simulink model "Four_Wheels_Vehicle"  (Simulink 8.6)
settings: Solver=ode45  StartTime=0.0  StopTime=20  RelTol=1e-3
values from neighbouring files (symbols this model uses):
  beta = 1    [Vehicle_Parameters.m]
  g = 9.81    [Vehicle_Parameters.m]
  H_CoG = 0.700    (= 0.7)    [Vehicle_Parameters.m]
  Hearo = 0.750    (= 0.75)    [Vehicle_Parameters.m]
  Iz = 2480    [Vehicle_Parameters.m]
  Jw = 2.166    [Vehicle_Parameters.m]
  L = 10    [Vehicle_Parameters.m]
  Lf = 1.180    (= 1.18)    [Vehicle_Parameters.m]
  Lr = 1.770    (= 1.77)    [Vehicle_Parameters.m]
  Lw = 1.880    (= 1.88)    [Vehicle_Parameters.m]
  m = 1500    [Vehicle_Parameters.m]
  miu = 0.85    [Vehicle_Parameters.m]
  reff = 0.380    (= 0.38)    [Vehicle_Parameters.m]
undefined symbols (not defined in the file or in its folder): DiscIntNeverNeededParam, Init, Ki, Kp, LowerLimit, sigbuilder_block, Ts, UpperLimit
libraries: simulink x15, powerlib_extras x3
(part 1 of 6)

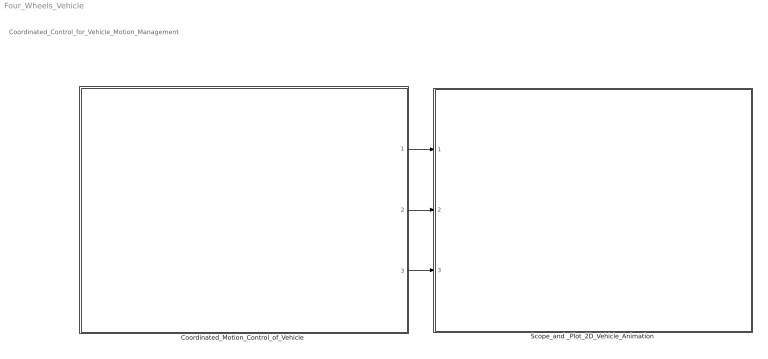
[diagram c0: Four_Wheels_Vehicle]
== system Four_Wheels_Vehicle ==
  note: Coordinated_Control_for_Vehicle_Motion_Management
  "Coordinated_Motion_Control_of_Vehicle " : Subsystem
  Scope_and _Plot_2D_Vehicle_Animation : Subsystem
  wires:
  "Coordinated_Motion_Control_of_Vehicle "/2(Control_of_braking_without_steering_control) -> Scope_and _Plot_2D_Vehicle_Animation/2(Control_of_braking_without_steering_control)
  "Coordinated_Motion_Control_of_Vehicle "/1(Coordinated_motion_control_Steering+Braking) -> Scope_and _Plot_2D_Vehicle_Animation/1(Coordinated_motion_control_Steering+Braking)
  "Coordinated_Motion_Control_of_Vehicle "/3(Control_of_steering_without_braking_control) -> Scope_and _Plot_2D_Vehicle_Animation/3(Control_of_steering_without_braking_control)

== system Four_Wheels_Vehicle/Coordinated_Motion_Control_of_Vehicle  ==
  Control_of_braking_without_steering_control. : Subsystem
  Control_of_steering_without_braking_control. : Subsystem
  Coordinated_motion_control_Steering+Braking. : Subsystem
  Mux : Mux  Inputs=8
  Mux1 : Mux  Inputs=8
  Mux2 : Mux  Inputs=8
  Coordinated_motion_control_Steering+Braking : Outport
  Control_of_braking_without_steering_control : Outport  Port=2
  Control_of_steering_without_braking_control : Outport  Port=3
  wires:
  Mux/1 -> Coordinated_motion_control_Steering+Braking/1
  Coordinated_motion_control_Steering+Braking./8(Ideal) -> Mux/8
  Coordinated_motion_control_Steering+Braking./6(yaw_pos.) -> Mux/6
  Coordinated_motion_control_Steering+Braking./7(SteeringAng) -> Mux/7
  Coordinated_motion_control_Steering+Braking./5(y_Vel) -> Mux/5
  Coordinated_motion_control_Steering+Braking./4(x_Vel) -> Mux/4
  Coordinated_motion_control_Steering+Braking./3(Tyre_speed) -> Mux/3
  Coordinated_motion_control_Steering+Braking./2(Estimated_trajectory) -> Mux/2
  Coordinated_motion_control_Steering+Braking./1(Ideal_trajectory) -> Mux/1
  Control_of_braking_without_steering_control./1(Ideal_trajectory_1) -> Mux1/1
  Control_of_braking_without_steering_control./2(Estimated_trajectory_1) -> Mux1/2
  Control_of_braking_without_steering_control./4(x_Vel_1) -> Mux1/4
  Control_of_braking_without_steering_control./5(y_Vel_1) -> Mux1/5
  Control_of_braking_without_steering_control./6(yaw_pos_1) -> Mux1/6
  Control_of_braking_without_steering_control./7(SteeringAng_1) -> Mux1/7
  Control_of_braking_without_steering_control./8(Ideal_1) -> Mux1/8
  Mux1/1 -> Control_of_braking_without_steering_control/1
  Control_of_steering_without_braking_control./1(Ideal_trajectory) -> Mux2/1
  Control_of_steering_without_braking_control./2(Estimated_trajectory) -> Mux2/2
  Control_of_steering_without_braking_control./3(Tyre_speed) -> Mux2/3
  Control_of_steering_without_braking_control./4(x_Vel) -> Mux2/4
  Control_of_steering_without_braking_control./5(y_Vel) -> Mux2/5
  Control_of_steering_without_braking_control./6(yaw_pos_2) -> Mux2/6
  Control_of_steering_without_braking_control./7(SteeringAng) -> Mux2/7
  Control_of_steering_without_braking_control./8(Ideal) -> Mux2/8
  Mux2/1 -> Control_of_steering_without_braking_control/1
  Control_of_braking_without_steering_control./3(Tyre_speed_1) -> Mux1/3

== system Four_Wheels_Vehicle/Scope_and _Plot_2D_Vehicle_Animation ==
  Coordinated_motion_control_Steering+Braking : Inport
  Control_of_braking_without_steering_control : Inport  Port=2
  Control_of_steering_without_braking_control : Inport  Port=3
  Scope_and _Plot_2D_Vehicle_Animation : Subsystem
  Signal_arrangement : Subsystem
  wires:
  Coordinated_motion_control_Steering+Braking/1 -> Signal_arrangement/1(Coordinated_motion_control_Steering+Braking)
  Control_of_braking_without_steering_control/1 -> Signal_arrangement/2(Control_of_braking_without_steering_control)
  Control_of_steering_without_braking_control/1 -> Signal_arrangement/3(Control_of_steering_without_braking_control)
  Signal_arrangement/1(Ideal_trajectory) -> Scope_and _Plot_2D_Vehicle_Animation/1(Ideal_trajectory)
  Signal_arrangement/2(Estimated_trajectory) -> Scope_and _Plot_2D_Vehicle_Animation/2(Estimated_trajectory)
  Signal_arrangement/3(Speed) -> Scope_and _Plot_2D_Vehicle_Animation/3(Speed)
  Signal_arrangement/4(Ideal_trajectory_1) -> Scope_and _Plot_2D_Vehicle_Animation/4(Ideal_trajectory_1)
  Signal_arrangement/5(Estimated_trajectory_1) -> Scope_and _Plot_2D_Vehicle_Animation/5(Estimated_trajectory_1)
  Signal_arrangement/6(Speed_1) -> Scope_and _Plot_2D_Vehicle_Animation/6(Speed_1)
  Signal_arrangement/7(Ideal_trajectory_2) -> Scope_and _Plot_2D_Vehicle_Animation/7(Ideal_trajectory_2)
  Signal_arrangement/8(Estimated_trajectory_2) -> Scope_and _Plot_2D_Vehicle_Animation/8(Estimated_trajectory_2)
  Signal_arrangement/9(Speed_2) -> Scope_and _Plot_2D_Vehicle_Animation/9(Speed_2)

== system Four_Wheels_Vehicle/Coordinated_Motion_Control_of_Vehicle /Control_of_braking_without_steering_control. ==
  note: Control_of_braking_without_steering_control
  Driver_command_1 : Subsystem
  Full_Vehicle_and_Tyre_Models_1 : Subsystem
  Motion_Coordinator_1 : Subsystem
  Scopes_and_2Dvehicle_1 : Subsystem
  Ideal_trajectory_1 : Outport
  Estimated_trajectory_1 : Outport  Port=2
  Tyre_speed_1 : Outport  Port=3
  x_Vel_1 : Outport  Port=4
  y_Vel_1 : Outport  Port=5
  yaw_pos_1 : Outport  Port=6
  SteeringAng_1 : Outport  Port=7
  Ideal_1 : Outport  Port=8
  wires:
  Motion_Coordinator_1/1(Ideal_traj._1) -> Scopes_and_2Dvehicle_1/2(Ideal._1)
  Scopes_and_2Dvehicle_1/8(Ideal_1) -> Ideal_1/1
  Scopes_and_2Dvehicle_1/7(SteeringAng_1) -> SteeringAng_1/1
  Scopes_and_2Dvehicle_1/5(y_Vel_1) -> y_Vel_1/1
  Scopes_and_2Dvehicle_1/4(x_Vel_1) -> x_Vel_1/1
  Scopes_and_2Dvehicle_1/2(Estimated_trajectory_1) -> Estimated_trajectory_1/1
  Scopes_and_2Dvehicle_1/1(Ideal_trajectory_1) -> Ideal_trajectory_1/1
  Driver_command_1/1(Steering_Ang._1) -> Motion_Coordinator_1/1(Steering_Ang_1), Scopes_and_2Dvehicle_1/1(SteeringAng._1)
  Full_Vehicle_and_Tyre_Models_1/2(x_Vel_1) -> Scopes_and_2Dvehicle_1/4(x_Vel._1), Motion_Coordinator_1/2(x_Vel)
  Full_Vehicle_and_Tyre_Models_1/5(yaw_rate_1) -> Motion_Coordinator_1/4(yaw_feedback_1), Scopes_and_2Dvehicle_1/7(yaw_rate._1)
  Full_Vehicle_and_Tyre_Models_1/4(sideslip_angle_1) -> Motion_Coordinator_1/3(Sideslip_feedback_1), Scopes_and_2Dvehicle_1/6(sideslipAng_1)
  Motion_Coordinator_1/2(f_1) -> Full_Vehicle_and_Tyre_Models_1/1(SteeringAng_1)
  Motion_Coordinator_1/3(Mzc_all_1) -> Full_Vehicle_and_Tyre_Models_1/2(Mzc_all_1)
  Full_Vehicle_and_Tyre_Models_1/3(y_Vel_1) -> Scopes_and_2Dvehicle_1/5(y_Vel._1)
  Motion_Coordinator_1/4(yaw_pos._1) -> yaw_pos_1/1
  Full_Vehicle_and_Tyre_Models_1/1(Tyre_speed_1) -> Scopes_and_2Dvehicle_1/3(Tyre_speed_1)
  Scopes_and_2Dvehicle_1/3(Tyre_speed_1.) -> Tyre_speed_1/1

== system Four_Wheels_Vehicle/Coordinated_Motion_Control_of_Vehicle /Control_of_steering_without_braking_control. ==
  note: Control_of_steering_without_braking_control
  Driver_command_2 : Subsystem
  Full_Vehicle_and_Tyre_Models_2 : Subsystem
  Motion_Coordinator_2 : Subsystem
  Scopes_and_2Dvehicle_2 : Subsystem
  Ideal_trajectory : Outport
  Estimated_trajectory : Outport  Port=2
  Tyre_speed : Outport  Port=3
  x_Vel : Outport  Port=4
  y_Vel : Outport  Port=5
  yaw_pos_2 : Outport  Port=6
  SteeringAng : Outport  Port=7
  Ideal : Outport  Port=8
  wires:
  Driver_command_2/1(Steering_Ang._2) -> Scopes_and_2Dvehicle_2/1(SteeringAng._2), Motion_Coordinator_2/1(Steering_Ang_2)
  Scopes_and_2Dvehicle_2/1(Ideal_trajectory_2) -> Ideal_trajectory/1
  Scopes_and_2Dvehicle_2/2(Estimated_trajectory_2) -> Estimated_trajectory/1
  Scopes_and_2Dvehicle_2/4(x_Vel_2) -> x_Vel/1
  Scopes_and_2Dvehicle_2/5(y_Vel_2) -> y_Vel/1
  Scopes_and_2Dvehicle_2/7(SteeringAng_2) -> SteeringAng/1
  Scopes_and_2Dvehicle_2/8(Ideal_2) -> Ideal/1
  Motion_Coordinator_2/1(Ideal_traj._2) -> Scopes_and_2Dvehicle_2/2(Ideal._2)
  Full_Vehicle_and_Tyre_Models_2/5(sideslip_angle) -> Motion_Coordinator_2/4(Sideslip_feedback_2), Scopes_and_2Dvehicle_2/7(sideslipAng_2)
  Full_Vehicle_and_Tyre_Models_2/4(yaw_rate_2) -> Motion_Coordinator_2/3(yaw_feedback_2), Scopes_and_2Dvehicle_2/6(yaw_rate._2)
  Full_Vehicle_and_Tyre_Models_2/2(x_Vel_2) -> Motion_Coordinator_2/2(x_Vel_2), Scopes_and_2Dvehicle_2/4(x_Vel._2)
  Motion_Coordinator_2/2(f_2) -> Full_Vehicle_and_Tyre_Models_2/1(SteeringAng)
  Motion_Coordinator_2/3(Mzc_all_2) -> Full_Vehicle_and_Tyre_Models_2/2(Mzc_all_2)
  Full_Vehicle_and_Tyre_Models_2/3(y_Vel_2) -> Scopes_and_2Dvehicle_2/5(y_Vel._2)
  Motion_Coordinator_2/4(yaw_pos_2) -> yaw_pos_2/1
  Full_Vehicle_and_Tyre_Models_2/1(Tyre_speed_2) -> Scopes_and_2Dvehicle_2/3(Tyre_speed_2)
  Scopes_and_2Dvehicle_2/3(Tyre_speed_2.) -> Tyre_speed/1

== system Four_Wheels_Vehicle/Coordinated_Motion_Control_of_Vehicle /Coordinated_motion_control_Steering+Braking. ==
  note: Coordinated_motion_control_Steering+Braking
  Driver_command : Subsystem
  Full_Vehicle_and_Tyre_Models : Subsystem
  Motion_Coordinator : Subsystem
  Scopes_and_2Dvehicle : Subsystem
  Ideal_trajectory : Outport
  Estimated_trajectory : Outport  Port=2
  Tyre_speed : Outport  Port=3
  x_Vel : Outport  Port=4
  y_Vel : Outport  Port=5
  yaw_pos. : Outport  Port=6
  SteeringAng : Outport  Port=7
  Ideal : Outport  Port=8
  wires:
  Driver_command/1(Steering_Ang.) -> Motion_Coordinator/1(Steering_Ang), Scopes_and_2Dvehicle/1(SteeringAng.)
  Scopes_and_2Dvehicle/1(Ideal_trajectory) -> Ideal_trajectory/1
  Scopes_and_2Dvehicle/2(Estimated_trajectory) -> Estimated_trajectory/1
  Scopes_and_2Dvehicle/4(x_Vel) -> x_Vel/1
  Scopes_and_2Dvehicle/5(y_Vel) -> y_Vel/1
  Scopes_and_2Dvehicle/7(SteeringAng) -> SteeringAng/1
  Scopes_and_2Dvehicle/8(Ideal) -> Ideal/1
  Motion_Coordinator/1(Ideal_traj.) -> Scopes_and_2Dvehicle/2(Ideal.)
  Motion_Coordinator/4(yaw_position) -> yaw_pos./1
  Full_Vehicle_and_Tyre_Models/5(sideslip_angle) -> Motion_Coordinator/4(Sideslip_feedback), Scopes_and_2Dvehicle/7(sideslipAng)
  Full_Vehicle_and_Tyre_Models/4(yaw_rate) -> Motion_Coordinator/3(yaw_feedback), Scopes_and_2Dvehicle/6(yaw_rate.)
  Full_Vehicle_and_Tyre_Models/2(x_Vel) -> Motion_Coordinator/2(x_Vel), Scopes_and_2Dvehicle/4(x_Vel.)
  Motion_Coordinator/2(f) -> Full_Vehicle_and_Tyre_Models/1(StreeringAng)
  Motion_Coordinator/3(Mzc_all) -> Full_Vehicle_and_Tyre_Models/2(Mzc_all)
  Full_Vehicle_and_Tyre_Models/3(y_Vel) -> Scopes_and_2Dvehicle/5(y_Vel.)
  Full_Vehicle_and_Tyre_Models/1(Tyre_speed) -> Scopes_and_2Dvehicle/3(Tyre_speed)
  Scopes_and_2Dvehicle/3(Tyre_speed.) -> Tyre_speed/1

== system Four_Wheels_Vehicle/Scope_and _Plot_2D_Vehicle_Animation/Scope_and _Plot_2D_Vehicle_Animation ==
  Ideal_trajectory : Inport
  Estimated_trajectory : Inport  Port=2
  Speed : Inport  Port=3
  Ideal_trajectory_1 : Inport  Port=4
  Estimated_trajectory_1 : Inport  Port=5
  Speed_1 : Inport  Port=6
  Ideal_trajectory_2 : Inport  Port=7
  Estimated_trajectory_2 : Inport  Port=8
  Speed_2 : Inport  Port=9
  Scopes : Subsystem
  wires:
  Speed_2/1 -> Scopes/9(Speed_2)
  Speed/1 -> Scopes/3(Speed)
  Estimated_trajectory_2/1 -> Scopes/8(Estimated_trajectory_2)
  Ideal_trajectory_2/1 -> Scopes/7(Ideal_trajectory_2)
  Speed_1/1 -> Scopes/6(Speed_1)
  Estimated_trajectory/1 -> Scopes/2(Estimated_trajectory)
  Ideal_trajectory_1/1 -> Scopes/4(Ideal_trajectory_1)
  Ideal_trajectory/1 -> Scopes/1(Ideal_trajectory)
  Estimated_trajectory_1/1 -> Scopes/5(Estimated_trajectory_1)

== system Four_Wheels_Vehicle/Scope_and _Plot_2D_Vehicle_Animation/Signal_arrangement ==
  Coordinated_motion_control_Steering+Braking : Inport
  Control_of_braking_without_steering_control : Inport  Port=2
  Control_of_steering_without_braking_control : Inport  Port=3
  Demux : Demux  Outputs=8
  Demux1 : Demux  Outputs=8
  Demux2 : Demux  Outputs=8
  Ideal_trajectory : Outport
  Estimated_trajectory : Outport  Port=2
  Speed : Outport  Port=3
  Ideal_trajectory_1 : Outport  Port=4
  Estimated_trajectory_1 : Outport  Port=5
  Speed_1 : Outport  Port=6
  Ideal_trajectory_2 : Outport  Port=7
  Estimated_trajectory_2 : Outport  Port=8
  Speed_2 : Outport  Port=9
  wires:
  Coordinated_motion_control_Steering+Braking/1 -> Demux/1
  Control_of_braking_without_steering_control/1 -> Demux1/1
  Control_of_steering_without_braking_control/1 -> Demux2/1
  Demux/1 -> Ideal_trajectory/1
  Demux/2 -> Estimated_trajectory/1
  Demux/3 -> Speed/1
  Demux1/1 -> Ideal_trajectory_1/1
  Demux1/2 -> Estimated_trajectory_1/1
  Demux1/3 -> Speed_1/1
  Demux2/3 -> Speed_2/1
  Demux2/2 -> Estimated_trajectory_2/1
  Demux2/1 -> Ideal_trajectory_2/1

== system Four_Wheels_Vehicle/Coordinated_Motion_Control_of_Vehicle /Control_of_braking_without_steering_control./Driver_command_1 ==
  2D Lookup Table : Lookup2D  RowIndex=[-3,-2,-1,0,1,2,3]  ColumnIndex=[0,1,2,3,4,5,6]  Table=reshape([0,0,0,0,0,0,0,-1,-1,-1,0,1,1,1,-2,-2,-2,0,2,2,2,-3,-3,-3,0,3,3,3,-4,-4,-4,0,4,4,4,-5,-5,-5,0,5,5,5,-6,-6,-6,0,6,6,6],7,7)  LookUpMeth=Interpolation-Use End Values
  2D Lookup Table1 : Lookup2D  RowIndex=[-3,-2,-1,0,1,2,3]  ColumnIndex=[0,1,2,3,4,5,6]  Table=reshape([0,0,0,0,0,0,0,-1,-1,-1,0,1,1,1,-2,-2,-2,0,2,2,2,-3,-3,-3,0,3,3,3,-4,-4,-4,0,4,4,4,-5,-5,-5,0,5,5,5,-6,-6,-6,0,6,6,6],7,7)  LookUpMeth=Interpolation-Use End Values
  2D Lookup Table2 : Lookup2D  RowIndex=[-3,-2,-1,0,1,2,3]  ColumnIndex=[0,1,2,3,4,5,6]  Table=reshape([0,0,0,0,0,0,0,-1,-1,-1,0,1,1,1,-2,-2,-2,0,2,2,2,-3,-3,-3,0,3,3,3,-4,-4,-4,0,4,4,4,-5,-5,-5,0,5,5,5,-6,-6,-6,0,6,6,6],7,7)  LookUpMeth=Interpolation-Use End Values  OutDataTypeStr=Inherit: Inherit via back propagation
  Controller : Subsystem
  Driver Torque : Sin  Frequency=0.4  SampleTime=0
  Driver Torque1 : Sin  Amplitude=4  Frequency=0.4  SampleTime=0
  Driver Torque2 : Sin  Frequency=0.6  SampleTime=0
  Driver Torque3 : Sin  Amplitude=2  Frequency=0.3  SampleTime=0
  Driver Torque4 : Sin  Frequency=0.4  SampleTime=1e-3
  Driver Torque5 : Sin  Amplitude=6  Frequency=0.2  SampleTime=1e-3
  Gain : Gain  Gain=1.29
  Gain1 : Gain  Gain=1/12
  Gain2 : Gain  Gain=1.7086
  Signal Builder1 : Subsystem  Tag=STV Subsys  LoadFcn=sigbuilder_block('load');  StartFcn=sigbuilder_block('start');  StopFcn=sigbuilder_block('stop');  ClipboardFcn=sigbuilder_block('clipboard');
  Steering_Ang : Constant  Value=20
  Steering_Angle1 : Subsystem  Tag=STV Subsys  LoadFcn=sigbuilder_block('load');  StartFcn=sigbuilder_block('start');  StopFcn=sigbuilder_block('stop');  ClipboardFcn=sigbuilder_block('clipboard');
  Steering_Dynamics : Subsystem
  Subsystem : Subsystem
  Transport Delay : TransportDelay  DelayTime=2  BufferSize=2048
  Transport Delay1 : TransportDelay  DelayTime=6  BufferSize=2048
  Transport Delay4 : TransportDelay  BufferSize=2048
  Transport Delay5 : TransportDelay  BufferSize=2048
  conv : Gain  Gain=(1/27.2957795)
  steering : ManualSwitch
  steering options : Subsystem
  swaDeg : Scope
  swaDeg1 : Scope  NumInputPorts=2
  swaDeg2 : Scope
  swaRad : Scope
  swaRad1 : Scope
  swaRad2 : Scope
  Steering_Ang._1 : Outport
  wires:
  steering options/1(delta_steer (rad)) -> swaDeg2/1
  Controller/1(Td (N-m)) -> Steering_Dynamics/1(Driver Torque)
  Steering_Dynamics/1(Steering Wheel Angle) -> Controller/1(Feedback), swaDeg1/2, Gain2/1
  2D Lookup Table/1 -> swaRad1/1
  Steering_Angle1/1(Imported_Signal 1) -> Gain1/1
  Transport Delay5/1 -> 2D Lookup Table2/2
  Driver Torque4/1 -> Transport Delay4/1
  Driver Torque5/1 -> Transport Delay5/1
  Transport Delay4/1 -> 2D Lookup Table2/1
  Transport Delay/1 -> 2D Lookup Table/1
  Driver Torque/1 -> Transport Delay/1
  Transport Delay1/1 -> 2D Lookup Table/2
  Driver Torque1/1 -> Transport Delay1/1
  conv/1 -> steering/1
  Gain2/1 -> swaDeg/1, conv/1
  steering/1 -> swaRad/1, Steering_Ang._1/1
  Steering_Ang/1 -> steering/2
  Driver Torque2/1 -> 2D Lookup Table1/1
  Driver Torque3/1 -> 2D Lookup Table1/2
  2D Lookup Table1/1 -> Gain/1
  Gain/1 -> swaRad2/1, Controller/2(Reference), swaDeg1/1

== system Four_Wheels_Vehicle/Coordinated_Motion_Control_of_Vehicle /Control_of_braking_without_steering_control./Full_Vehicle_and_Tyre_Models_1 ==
  SteeringAng_1 : Inport
  Mzc_all_1 : Inport  Port=2
  Tyre_model_1 : Subsystem
  Vehicle_body_1 : Subsystem
  Tyre_speed_1 : Outport
  x_Vel_1 : Outport  Port=2
  y_Vel_1 : Outport  Port=3
  sideslip_angle_1 : Outport  Port=4
  yaw_rate_1 : Outport  Port=5
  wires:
  SteeringAng_1/1 -> Tyre_model_1/1(SteeringAng_1), Vehicle_body_1/1(Steering_Ang._1)
  Mzc_all_1/1 -> Tyre_model_1/4(Mzc_all_1)
  Tyre_model_1/2(Fx_and_Fy_1) -> Vehicle_body_1/2(Fx_and_Fy_1)
  Tyre_model_1/1(Tyre_rotational_speed_1) -> Tyre_speed_1/1
  Vehicle_body_1/4(side-slip angle_1) -> Tyre_model_1/6(beta), sideslip_angle_1/1
  Vehicle_body_1/3(yaw_rate_1) -> Tyre_model_1/5(yaw_rate_1), yaw_rate_1/1
  Vehicle_body_1/1(x_Vel_1) -> x_Vel_1/1, Tyre_model_1/2(x_Vel_1)
  Vehicle_body_1/2(y_Vel_1) -> y_Vel_1/1, Tyre_model_1/3(y_Vel_1)

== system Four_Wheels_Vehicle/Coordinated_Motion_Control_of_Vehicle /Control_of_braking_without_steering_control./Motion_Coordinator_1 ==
  Steering_Ang_1 : Inport
  x_Vel : Inport  Port=2
  Sideslip_feedback_1 : Inport  Port=3
  yaw_feedback_1 : Inport  Port=4
  Constant_speed_1 (m/s) : Constant  Value=5
  Controller_and_actuator Steering_and_Braking_1 : Subsystem
  Coordinate_Transformation_Model_1 : Subsystem
  Gain1 : Gain  Gain=10
  Gain2 : Gain
  Ideal_trajetory_1 : Subsystem
  Mux : Mux
  Sideslip_angle6 : Scope  NumInputPorts=2
  x_seitch : ManualSwitch  CurrentSetting=0
  Ideal_traj._1 : Outport
  f_1 : Outport  Port=2
  Mzc_all_1 : Outport  Port=3
  yaw_pos._1 : Outport  Port=4
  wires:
  Mux/1 -> Mzc_all_1/1
  Controller_and_actuator Steering_and_Braking_1/2(Mzc_1) -> Mux/1
  Controller_and_actuator Steering_and_Braking_1/3(Mzc_2) -> Mux/2
  Controller_and_actuator Steering_and_Braking_1/4(Mzc_3) -> Mux/3
  Controller_and_actuator Steering_and_Braking_1/5(Mzc_4) -> Mux/4
  Gain2/1 -> Controller_and_actuator Steering_and_Braking_1/1(StteringAng)
  Ideal_trajetory_1/1(Y-position) -> Ideal_traj._1/1
  Coordinate_Transformation_Model_1/2(Y-position) -> Sideslip_angle6/2
  Coordinate_Transformation_Model_1/1(X-position) -> Sideslip_angle6/1
  Controller_and_actuator Steering_and_Braking_1/1(f) -> f_1/1
  Sideslip_feedback_1/1 -> Controller_and_actuator Steering_and_Braking_1/5(Feedback_Sideslip)
  Coordinate_Transformation_Model_1/4(Sideslip_beta) -> Controller_and_actuator Steering_and_Braking_1/3(Reference_Sideslip)
  Coordinate_Transformation_Model_1/3(yaw_Rate) -> Controller_and_actuator Steering_and_Braking_1/2(Reference_Steering)
  yaw_feedback_1/1 -> Controller_and_actuator Steering_and_Braking_1/4(Feedback_Steering)
  Steering_Ang_1/1 -> Gain2/1, Gain1/1, Ideal_trajetory_1/1(SteeringAng)
  x_Vel/1 -> x_seitch/2
  Gain1/1 -> Coordinate_Transformation_Model_1/1(delta_steer (rad))
  Constant_speed_1 (m/s)/1 -> x_seitch/1
  x_seitch/1 -> Coordinate_Transformation_Model_1/2(v_x (m/s))
  Coordinate_Transformation_Model_1/5(yaw_pos.) -> yaw_pos._1/1

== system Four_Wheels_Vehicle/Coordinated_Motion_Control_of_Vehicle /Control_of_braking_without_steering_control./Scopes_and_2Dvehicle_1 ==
  SteeringAng._1 : Inport
  Ideal._1 : Inport  Port=2
  Tyre_speed_1 : Inport  Port=3
  x_Vel._1 : Inport  Port=4
  y_Vel._1 : Inport  Port=5
  sideslipAng_1 : Inport  Port=6
  yaw_rate._1 : Inport  Port=7
  Scopes_1 : Subsystem
  Signals_to_2Dvehicle_1 : Subsystem
  Ideal_trajectory_1 : Outport
  Estimated_trajectory_1 : Outport  Port=2
  Tyre_speed_1. : Outport  Port=3
  x_Vel_1 : Outport  Port=4
  y_Vel_1 : Outport  Port=5
  yaw_rate_1 : Outport  Port=6
  SteeringAng_1 : Outport  Port=7
  Ideal_1 : Outport  Port=8
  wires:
  Ideal._1/1 -> Signals_to_2Dvehicle_1/5(Ideal._1), Scopes_1/6(Ideal_1)
  sideslipAng_1/1 -> Scopes_1/5(sideslipAng_1)
  yaw_rate._1/1 -> Scopes_1/4(yaw_rate_1), Signals_to_2Dvehicle_1/4(yaw_rate._1)
  y_Vel._1/1 -> Signals_to_2Dvehicle_1/3(y_Vel._1), Scopes_1/3(y_Vel_1)
  x_Vel._1/1 -> Scopes_1/2(x_Vel_1), Signals_to_2Dvehicle_1/2(x_Vel._1)
  SteeringAng._1/1 -> Scopes_1/1(SteeringAng_1), Signals_to_2Dvehicle_1/1(SteeringAng._1)
  Signals_to_2Dvehicle_1/4(SteeringAng_1) -> SteeringAng_1/1
  Signals_to_2Dvehicle_1/5(Ideal_1) -> Ideal_1/1
  Signals_to_2Dvehicle_1/1(x_Vel_1) -> x_Vel_1/1
  Signals_to_2Dvehicle_1/2(y_Vel_1) -> y_Vel_1/1
  Signals_to_2Dvehicle_1/3(yaw_rate_1) -> yaw_rate_1/1
  Scopes_1/2(Estimated_trajectory_1) -> Estimated_trajectory_1/1
  Scopes_1/1(Ideal_trajectory_1) -> Ideal_trajectory_1/1
  Tyre_speed_1/1 -> Tyre_speed_1./1

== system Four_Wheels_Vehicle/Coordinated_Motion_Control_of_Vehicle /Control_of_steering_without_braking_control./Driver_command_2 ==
  2D Lookup Table : Lookup2D  RowIndex=[-3,-2,-1,0,1,2,3]  ColumnIndex=[0,1,2,3,4,5,6]  Table=reshape([0,0,0,0,0,0,0,-1,-1,-1,0,1,1,1,-2,-2,-2,0,2,2,2,-3,-3,-3,0,3,3,3,-4,-4,-4,0,4,4,4,-5,-5,-5,0,5,5,5,-6,-6,-6,0,6,6,6],7,7)  LookUpMeth=Interpolation-Use End Values
  2D Lookup Table1 : Lookup2D  RowIndex=[-3,-2,-1,0,1,2,3]  ColumnIndex=[0,1,2,3,4,5,6]  Table=reshape([0,0,0,0,0,0,0,-1,-1,-1,0,1,1,1,-2,-2,-2,0,2,2,2,-3,-3,-3,0,3,3,3,-4,-4,-4,0,4,4,4,-5,-5,-5,0,5,5,5,-6,-6,-6,0,6,6,6],7,7)  LookUpMeth=Interpolation-Use End Values
  2D Lookup Table2 : Lookup2D  RowIndex=[-3,-2,-1,0,1,2,3]  ColumnIndex=[0,1,2,3,4,5,6]  Table=reshape([0,0,0,0,0,0,0,-1,-1,-1,0,1,1,1,-2,-2,-2,0,2,2,2,-3,-3,-3,0,3,3,3,-4,-4,-4,0,4,4,4,-5,-5,-5,0,5,5,5,-6,-6,-6,0,6,6,6],7,7)  LookUpMeth=Interpolation-Use End Values  OutDataTypeStr=Inherit: Inherit via back propagation
  Controller : Subsystem
  Driver Torque : Sin  Frequency=0.4  SampleTime=0
  Driver Torque1 : Sin  Amplitude=4  Frequency=0.4  SampleTime=0
  Driver Torque2 : Sin  Frequency=0.6  SampleTime=0
  Driver Torque3 : Sin  Amplitude=2  Frequency=0.3  SampleTime=0
  Driver Torque4 : Sin  Frequency=0.4  SampleTime=1e-3
  Driver Torque5 : Sin  Amplitude=6  Frequency=0.2  SampleTime=1e-3
  Gain : Gain  Gain=1.1
  Gain1 : Gain  Gain=1/12
  Gain2 : Gain  Gain=1.7086
  Signal Builder1 : Subsystem  Tag=STV Subsys  LoadFcn=sigbuilder_block('load');  StartFcn=sigbuilder_block('start');  StopFcn=sigbuilder_block('stop');  ClipboardFcn=sigbuilder_block('clipboard');
  Steering_Ang : Constant  Value=20
  Steering_Angle1 : Subsystem  Tag=STV Subsys  LoadFcn=sigbuilder_block('load');  StartFcn=sigbuilder_block('start');  StopFcn=sigbuilder_block('stop');  ClipboardFcn=sigbuilder_block('clipboard');
  Steering_Dynamics : Subsystem
  Subsystem : Subsystem
  Transport Delay : TransportDelay  DelayTime=2  BufferSize=2048
  Transport Delay1 : TransportDelay  DelayTime=6  BufferSize=2048
  Transport Delay4 : TransportDelay  BufferSize=2048
  Transport Delay5 : TransportDelay  BufferSize=2048
  conv : Gain  Gain=(1/27.2957795)
  steering : ManualSwitch
  steering options : Subsystem
  swaDeg : Scope
  swaDeg1 : Scope  NumInputPorts=2
  swaDeg2 : Scope
  swaDeg4 : Scope
  swaRad : Scope
  swaRad1 : Scope
  swaRad2 : Scope
  Steering_Ang._2 : Outport
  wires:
  Steering_Ang/1 -> steering/2
  steering/1 -> Steering_Ang._2/1, swaRad/1
  Gain2/1 -> conv/1, swaDeg/1
  conv/1 -> steering/1
  Driver Torque1/1 -> Transport Delay1/1
  Transport Delay1/1 -> 2D Lookup Table/2
  Driver Torque/1 -> Transport Delay/1
  Transport Delay/1 -> 2D Lookup Table/1
  Transport Delay4/1 -> 2D Lookup Table2/1
  Driver Torque5/1 -> Transport Delay5/1
  Driver Torque4/1 -> Transport Delay4/1
  Transport Delay5/1 -> 2D Lookup Table2/2
  Steering_Angle1/1(Imported_Signal 1) -> Gain1/1
  2D Lookup Table/1 -> swaRad1/1
  Steering_Dynamics/1(Steering Wheel Angle) -> Gain2/1, swaDeg1/2, Controller/1(Feedback)
  Controller/1(Td (N-m)) -> Steering_Dynamics/1(Driver Torque)
  steering options/1(delta_steer (rad)) -> swaDeg2/1
  2D Lookup Table2/1 -> swaDeg4/1
  Driver Torque2/1 -> 2D Lookup Table1/1
  Driver Torque3/1 -> 2D Lookup Table1/2
  2D Lookup Table1/1 -> Gain/1
  Gain/1 -> swaRad2/1, swaDeg1/1, Controller/2(Reference)

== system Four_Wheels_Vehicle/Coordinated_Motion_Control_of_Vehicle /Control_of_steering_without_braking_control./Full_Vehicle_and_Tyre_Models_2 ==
  SteeringAng : Inport
  Mzc_all_2 : Inport  Port=2
  Tyre_model_2 : Subsystem
  Vehicle_body_2 : Subsystem
  Tyre_speed_2 : Outport
  x_Vel_2 : Outport  Port=2
  y_Vel_2 : Outport  Port=3
  yaw_rate_2 : Outport  Port=4
  sideslip_angle : Outport  Port=5
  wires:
  Vehicle_body_2/2(y_Vel_2) -> y_Vel_2/1, Tyre_model_2/3(y_Vel_2)
  Vehicle_body_2/1(x_Vel_2) -> x_Vel_2/1, Tyre_model_2/2(x_Ve_2l)
  Vehicle_body_2/3(yaw_rate_2) -> Tyre_model_2/5(yaw_rate_2), yaw_rate_2/1
  Vehicle_body_2/4(side-slip angle_2) -> Tyre_model_2/6(beta_2), sideslip_angle/1
  Tyre_model_2/1(Tyre_rotational_speed) -> Tyre_speed_2/1
  Tyre_model_2/2(Fx_and_Fy_2) -> Vehicle_body_2/2(Fx_and_Fy_2)
  Mzc_all_2/1 -> Tyre_model_2/4(Mzc_all_2)
  SteeringAng/1 -> Tyre_model_2/1(SteeringAng_2), Vehicle_body_2/1(Steering_Ang._2)

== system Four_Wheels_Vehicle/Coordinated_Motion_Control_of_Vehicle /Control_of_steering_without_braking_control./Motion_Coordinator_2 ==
  Steering_Ang_2 : Inport
  x_Vel_2 : Inport  Port=2
  yaw_feedback_2 : Inport  Port=3
  Sideslip_feedback_2 : Inport  Port=4
  Constant_speed_2 (m/s) : Constant  Value=5
  Controller_and_actuator Steering_and_Braking_2 : Subsystem
  Coordinate_Transformation_Model_2 : Subsystem
  Gain1 : Gain  Gain=10
  Gain2 : Gain
  Ideal_trajetory_2 : Subsystem
  Mux : Mux
  Sideslip_angle6 : Scope  NumInputPorts=2
  x_seitch : ManualSwitch  CurrentSetting=0
  Ideal_traj._2 : Outport
  f_2 : Outport  Port=2
  Mzc_all_2 : Outport  Port=3
  yaw_pos_2 : Outport  Port=4
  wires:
  x_seitch/1 -> Coordinate_Transformation_Model_2/2(v_x (m/s))
  Constant_speed_2 (m/s)/1 -> x_seitch/1
  Gain1/1 -> Coordinate_Transformation_Model_2/1(delta_steer (rad))
  x_Vel_2/1 -> x_seitch/2
  Steering_Ang_2/1 -> Ideal_trajetory_2/1(SteeringAng), Gain1/1, Gain2/1
  yaw_feedback_2/1 -> Controller_and_actuator Steering_and_Braking_2/4(Feedback_Steering)
  Coordinate_Transformation_Model_2/3(yaw_Rate) -> Controller_and_actuator Steering_and_Braking_2/2(Reference_Steering)
  Coordinate_Transformation_Model_2/4(Sideslip_beta) -> Controller_and_actuator Steering_and_Braking_2/3(Reference_Sideslip)
  Sideslip_feedback_2/1 -> Controller_and_actuator Steering_and_Braking_2/5(Feedback_Sideslip)
  Controller_and_actuator Steering_and_Braking_2/1(f) -> f_2/1
  Coordinate_Transformation_Model_2/1(X-position) -> Sideslip_angle6/1
  Coordinate_Transformation_Model_2/2(Y-position) -> Sideslip_angle6/2
  Ideal_trajetory_2/1(Y-position) -> Ideal_traj._2/1
  Gain2/1 -> Controller_and_actuator Steering_and_Braking_2/1(StteringAng)
  Controller_and_actuator Steering_and_Braking_2/5(Mzc_4) -> Mux/4
  Controller_and_actuator Steering_and_Braking_2/4(Mzc_3) -> Mux/3
  Controller_and_actuator Steering_and_Braking_2/3(Mzc_2) -> Mux/2
  Controller_and_actuator Steering_and_Braking_2/2(Mzc_1) -> Mux/1
  Mux/1 -> Mzc_all_2/1
  Coordinate_Transformation_Model_2/5(yaw_pos._2) -> yaw_pos_2/1

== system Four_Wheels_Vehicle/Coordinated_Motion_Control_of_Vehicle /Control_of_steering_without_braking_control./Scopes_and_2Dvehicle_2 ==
  SteeringAng._2 : Inport
  Ideal._2 : Inport  Port=2
  Tyre_speed_2 : Inport  Port=3
  x_Vel._2 : Inport  Port=4
  y_Vel._2 : Inport  Port=5
  yaw_rate._2 : Inport  Port=6
  sideslipAng_2 : Inport  Port=7
  Scopes : Subsystem
  Signals_to_2Dvehicle : Subsystem
  Ideal_trajectory_2 : Outport
  Estimated_trajectory_2 : Outport  Port=2
  Tyre_speed_2. : Outport  Port=3
  x_Vel_2 : Outport  Port=4
  y_Vel_2 : Outport  Port=5
  yaw_rate_2 : Outport  Port=6
  SteeringAng_2 : Outport  Port=7
  Ideal_2 : Outport  Port=8
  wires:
  Scopes/1(Ideal_trajectory_2) -> Ideal_trajectory_2/1
  Scopes/2(Estimated_trajectory_2) -> Estimated_trajectory_2/1
  Signals_to_2Dvehicle/3(yaw_rate_2) -> yaw_rate_2/1
  Signals_to_2Dvehicle/2(y_Vel_2) -> y_Vel_2/1
  Signals_to_2Dvehicle/1(x_Vel_2) -> x_Vel_2/1
  Signals_to_2Dvehicle/5(Ideal_2) -> Ideal_2/1
  Signals_to_2Dvehicle/4(SteeringAng_2) -> SteeringAng_2/1
  SteeringAng._2/1 -> Signals_to_2Dvehicle/1(SteeringAng._2), Scopes/1(SteeringAng_2)
  x_Vel._2/1 -> Signals_to_2Dvehicle/2(x_Vel._2), Scopes/2(x_Vel_2)
  y_Vel._2/1 -> Scopes/3(y_Vel_2), Signals_to_2Dvehicle/3(y_Vel._2)
  yaw_rate._2/1 -> Signals_to_2Dvehicle/4(yaw_rate._2), Scopes/4(yaw_rate_2)
  sideslipAng_2/1 -> Scopes/5(sideslipAng_2)
  Ideal._2/1 -> Scopes/6(Ideal_2), Signals_to_2Dvehicle/5(Ideal._2)
  Tyre_speed_2/1 -> Tyre_speed_2./1

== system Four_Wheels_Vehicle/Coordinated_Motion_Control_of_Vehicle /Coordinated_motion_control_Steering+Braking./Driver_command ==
  2D Lookup Table : Lookup2D  RowIndex=[-3,-2,-1,0,1,2,3]  ColumnIndex=[0,1,2,3,4,5,6]  Table=reshape([0,0,0,0,0,0,0,-1,-1,-1,0,1,1,1,-2,-2,-2,0,2,2,2,-3,-3,-3,0,3,3,3,-4,-4,-4,0,4,4,4,-5,-5,-5,0,5,5,5,-6,-6,-6,0,6,6,6],7,7)  LookUpMeth=Interpolation-Use End Values
  2D Lookup Table1 : Lookup2D  RowIndex=[-3,-2,-1,0,1,2,3]  ColumnIndex=[0,1,2,3,4,5,6]  Table=reshape([0,0,0,0,0,0,0,-1,-1,-1,0,1,1,1,-2,-2,-2,0,2,2,2,-3,-3,-3,0,3,3,3,-4,-4,-4,0,4,4,4,-5,-5,-5,0,5,5,5,-6,-6,-6,0,6,6,6],7,7)  LookUpMeth=Interpolation-Use End Values
  2D Lookup Table2 : Lookup2D  RowIndex=[-3,-2,-1,0,1,2,3]  ColumnIndex=[0,1,2,3,4,5,6]  Table=reshape([0,0,0,0,0,0,0,-1,-1,-1,0,1,1,1,-2,-2,-2,0,2,2,2,-3,-3,-3,0,3,3,3,-4,-4,-4,0,4,4,4,-5,-5,-5,0,5,5,5,-6,-6,-6,0,6,6,6],7,7)  LookUpMeth=Interpolation-Use End Values  OutDataTypeStr=Inherit: Inherit via back propagation
  Controller : Subsystem
  Driver Torque : Sin  Frequency=0.4  SampleTime=0
  Driver Torque1 : Sin  Amplitude=4  Frequency=0.4  SampleTime=0
  Driver Torque2 : Sin  Frequency=0.6  SampleTime=0
  Driver Torque3 : Sin  Amplitude=2  Frequency=0.3  SampleTime=0
  Driver Torque4 : Sin  Frequency=0.4  SampleTime=1e-3
  Driver Torque5 : Sin  Amplitude=6  Frequency=0.2  SampleTime=1e-3
  Gain : Gain  Gain=1.29
  Gain1 : Gain  Gain=1/12
  Gain2 : Gain  Gain=1.7086
  Signal Builder1 : Subsystem  Tag=STV Subsys  LoadFcn=sigbuilder_block('load');  StartFcn=sigbuilder_block('start');  StopFcn=sigbuilder_block('stop');  ClipboardFcn=sigbuilder_block('clipboard');
  Steering_Ang : Constant  Value=20
  Steering_Angle1 : Subsystem  Tag=STV Subsys  LoadFcn=sigbuilder_block('load');  StartFcn=sigbuilder_block('start');  StopFcn=sigbuilder_block('stop');  ClipboardFcn=sigbuilder_block('clipboard');
  Steering_Dynamics : Subsystem
  Subsystem : Subsystem
  Transport Delay : TransportDelay  DelayTime=2  BufferSize=2048
  Transport Delay1 : TransportDelay  DelayTime=6  BufferSize=2048
  Transport Delay4 : TransportDelay  BufferSize=2048
  Transport Delay5 : TransportDelay  BufferSize=2048
  conv : Gain  Gain=(1/27.2957795)
  steering : ManualSwitch
  steering options : Subsystem
  swaDeg : Scope
  swaDeg1 : Scope  NumInputPorts=2
  swaDeg2 : Scope
  swaRad : Scope
  swaRad1 : Scope
  swaRad2 : Scope
  swaRad3 : Scope  NumInputPorts=2
  Steering_Ang. : Outport
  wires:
  Steering_Ang/1 -> steering/2
  steering/1 -> Steering_Ang./1, swaRad/1
  Gain2/1 -> conv/1, swaDeg/1
  conv/1 -> steering/1
  Driver Torque2/1 -> 2D Lookup Table1/1
  Driver Torque3/1 -> 2D Lookup Table1/2
  Driver Torque1/1 -> Transport Delay1/1
  Transport Delay1/1 -> 2D Lookup Table/2
  Driver Torque/1 -> Transport Delay/1
  Transport Delay4/1 -> 2D Lookup Table2/1
  Driver Torque5/1 -> Transport Delay5/1
  Driver Torque4/1 -> Transport Delay4/1
  Transport Delay5/1 -> 2D Lookup Table2/2
  Steering_Angle1/1(Imported_Signal 1) -> Gain1/1
  Steering_Dynamics/1(Steering Wheel Angle) -> swaRad3/1, Gain2/1, swaDeg1/2, Controller/1(Feedback)
  Controller/1(Td (N-m)) -> Steering_Dynamics/1(Driver Torque)
  steering options/1(delta_steer (rad)) -> swaDeg2/1
  2D Lookup Table/1 -> swaRad1/1
  Transport Delay/1 -> 2D Lookup Table/1
  2D Lookup Table1/1 -> Gain/1
  Gain/1 -> Controller/2(Reference), swaRad2/1
  Steering_Dynamics/2(Ts) -> swaRad3/2

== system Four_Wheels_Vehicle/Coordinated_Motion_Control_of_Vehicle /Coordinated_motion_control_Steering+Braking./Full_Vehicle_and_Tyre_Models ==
  StreeringAng : Inport
  Mzc_all : Inport  Port=2
  Tyre_model : Subsystem
  Vehicle_body : Subsystem
  Tyre_speed : Outport
  x_Vel : Outport  Port=2
  y_Vel : Outport  Port=3
  yaw_rate : Outport  Port=4
  sideslip_angle : Outport  Port=5
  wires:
  Vehicle_body/2(y_Vel) -> y_Vel/1, Tyre_model/3(y_Vel)
  Vehicle_body/1(x_Vel) -> x_Vel/1, Tyre_model/2(x_Vel)
  Vehicle_body/3(yaw_rate) -> yaw_rate/1, Tyre_model/5(yaw_rate)
  Vehicle_body/4(side-slip angle) -> sideslip_angle/1, Tyre_model/6(beta)
  Tyre_model/1(Tyre_rotational_speed) -> Tyre_speed/1
  Tyre_model/2(Fx_and_Fy) -> Vehicle_body/2(Fx_and_Fy)
  Mzc_all/1 -> Tyre_model/4(Mzc_all)
  StreeringAng/1 -> Vehicle_body/1(Steering_Ang.), Tyre_model/1(SteeringAng)

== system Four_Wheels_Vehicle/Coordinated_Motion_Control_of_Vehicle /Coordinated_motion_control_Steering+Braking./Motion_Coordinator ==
  Steering_Ang : Inport
  x_Vel : Inport  Port=2
  yaw_feedback : Inport  Port=3
  Sideslip_feedback : Inport  Port=4
  Constant_speed (m/s) : Constant  Value=5
  Controller_and_actuator Steering_and_Braking : Subsystem
  Coordinate_Transformation_Model : Subsystem
  Gain1 : Gain  Gain=10
  Gain2 : Gain
  Ideal_trajetory : Subsystem
  Mux : Mux
  Sideslip_angle6 : Scope  NumInputPorts=2
  x_seitch : ManualSwitch  CurrentSetting=0
  Ideal_traj. : Outport
  f : Outport  Port=2
  Mzc_all : Outport  Port=3
  yaw_position : Outport  Port=4
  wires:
  x_seitch/1 -> Coordinate_Transformation_Model/2(v_x (m/s))
  Constant_speed (m/s)/1 -> x_seitch/1
  Gain1/1 -> Coordinate_Transformation_Model/1(delta_steer (rad))
  x_Vel/1 -> x_seitch/2
  Steering_Ang/1 -> Ideal_trajetory/1(SteeringAng), Gain1/1, Gain2/1
  yaw_feedback/1 -> Controller_and_actuator Steering_and_Braking/4(Feedback_Steering)
  Coordinate_Transformation_Model/3(yaw_Rate) -> Controller_and_actuator Steering_and_Braking/2(Reference_Steering)
  Coordinate_Transformation_Model/4(Sideslip_beta) -> Controller_and_actuator Steering_and_Braking/3(Reference_Sideslip)
  Sideslip_feedback/1 -> Controller_and_actuator Steering_and_Braking/5(Feedback_Sideslip)
  Controller_and_actuator Steering_and_Braking/1(f) -> f/1
  Coordinate_Transformation_Model/1(X-position) -> Sideslip_angle6/1
  Coordinate_Transformation_Model/2(Y-position) -> Sideslip_angle6/2
  Ideal_trajetory/1(Y-position) -> Ideal_traj./1
  Gain2/1 -> Controller_and_actuator Steering_and_Braking/1(StteringAng)
  Controller_and_actuator Steering_and_Braking/5(Mzc_4) -> Mux/4
  Controller_and_actuator Steering_and_Braking/4(Mzc_3) -> Mux/3
  Controller_and_actuator Steering_and_Braking/3(Mzc_2) -> Mux/2
  Controller_and_actuator Steering_and_Braking/2(Mzc_1) -> Mux/1
  Mux/1 -> Mzc_all/1
  Coordinate_Transformation_Model/5(yaw_position) -> yaw_position/1

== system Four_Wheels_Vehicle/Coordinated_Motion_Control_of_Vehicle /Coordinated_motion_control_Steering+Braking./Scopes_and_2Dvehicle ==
  SteeringAng. : Inport
  Ideal. : Inport  Port=2
  Tyre_speed : Inport  Port=3
  x_Vel. : Inport  Port=4
  y_Vel. : Inport  Port=5
  yaw_rate. : Inport  Port=6
  sideslipAng : Inport  Port=7
  Scopes : Subsystem
  Signals_to_2Dvehicle : Subsystem
  Ideal_trajectory : Outport
  Estimated_trajectory : Outport  Port=2
  Tyre_speed. : Outport  Port=3
  x_Vel : Outport  Port=4
  y_Vel : Outport  Port=5
  yaw_rate : Outport  Port=6
  SteeringAng : Outport  Port=7
  Ideal : Outport  Port=8
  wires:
  Scopes/1(Ideal_trajectory) -> Ideal_trajectory/1
  Scopes/2(Estimated_trajectory) -> Estimated_trajectory/1
  Signals_to_2Dvehicle/3(yaw_rate) -> yaw_rate/1
  Signals_to_2Dvehicle/2(y_Vel) -> y_Vel/1
  Signals_to_2Dvehicle/1(x_Vel) -> x_Vel/1
  Signals_to_2Dvehicle/5(Ideal) -> Ideal/1
  Signals_to_2Dvehicle/4(SteeringAng) -> SteeringAng/1
  SteeringAng./1 -> Signals_to_2Dvehicle/1(SteeringAng.), Scopes/1(SteeringAng)
  x_Vel./1 -> Signals_to_2Dvehicle/2(x_Vel.), Scopes/2(x_Vel)
  y_Vel./1 -> Scopes/3(y_Vel), Signals_to_2Dvehicle/3(y_Vel.)
  yaw_rate./1 -> Signals_to_2Dvehicle/4(yaw_rate.), Scopes/4(yaw_rate)
  sideslipAng/1 -> Scopes/5(sideslipAng)
  Ideal./1 -> Scopes/6(Ideal), Signals_to_2Dvehicle/5(Ideal.)
  Tyre_speed/1 -> Tyre_speed./1

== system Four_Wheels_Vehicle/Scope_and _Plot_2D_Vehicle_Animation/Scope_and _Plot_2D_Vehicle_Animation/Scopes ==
  Ideal_trajectory : Inport
  Estimated_trajectory : Inport  Port=2
  Speed : Inport  Port=3
  Ideal_trajectory_1 : Inport  Port=4
  Estimated_trajectory_1 : Inport  Port=5
  Speed_1 : Inport  Port=6
  Ideal_trajectory_2 : Inport  Port=7
  Estimated_trajectory_2 : Inport  Port=8
  Speed_2 : Inport  Port=9
  Mux1 : Mux  Inputs=2
  Mux2 : Mux  Inputs=2
  Mux6 : Mux  Inputs=2
  Performance_Comparsion : Scope  NumInputPorts=3
  Performance_Comparsion tyre_rotational_speed : Scope  NumInputPorts=3
  Performance_Comparsion1 : Scope  NumInputPorts=4
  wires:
  Speed_1/1 -> Performance_Comparsion tyre_rotational_speed/2
  Speed_2/1 -> Performance_Comparsion tyre_rotational_speed/3
  Estimated_trajectory_2/1 -> Mux2/2, Performance_Comparsion1/4
  Estimated_trajectory_1/1 -> Mux1/2, Performance_Comparsion1/3
  Estimated_trajectory/1 -> Performance_Comparsion1/2, Mux6/2
  Speed/1 -> Performance_Comparsion tyre_rotational_speed/1
  Ideal_trajectory/1 -> Performance_Comparsion1/1, Mux6/1
  Mux2/1 -> Performance_Comparsion/3
  Mux6/1 -> Performance_Comparsion/1
  Mux1/1 -> Performance_Comparsion/2
  Ideal_trajectory_1/1 -> Mux1/1
  Ideal_trajectory_2/1 -> Mux2/1

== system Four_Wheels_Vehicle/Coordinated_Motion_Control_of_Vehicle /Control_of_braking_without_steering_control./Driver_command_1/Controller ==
  Feedback : Inport
  Reference : Inport  Port=2
  Controller : powerlib_extras/Discrete  Control Blocks/Discrete PI Controller  Kp=20  Ki=0.15  Par_Limits=[10 -10]  Init=0  Ts=800e-6
  Scope3 : Scope
  Sum1 : Sum  Inputs=-+
  Td (N-m) : Outport
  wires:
  Reference/1 -> Sum1/2
  Controller/1 -> Td (N-m)/1, Scope3/1
  Sum1/1 -> Controller/1
  Feedback/1 -> Sum1/1

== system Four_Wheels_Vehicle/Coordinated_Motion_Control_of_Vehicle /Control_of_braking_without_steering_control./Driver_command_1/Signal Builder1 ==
  Demux : Demux  Tag=STV Demux  Outputs=2
  FromWs : FromWorkspace  Tag=STV FromWs  VariableName=tuvar  SampleTime=0  SigBuilderData=DataTag0  VnvData=DataTag1
  Signal 1 : Outport  Tag=STV Outport
  Signal 2 : Outport  Tag=STV Outport  Port=2
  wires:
  Demux/1 -> Signal 1/1
  FromWs/1 -> Demux/1
  Demux/2 -> Signal 2/1

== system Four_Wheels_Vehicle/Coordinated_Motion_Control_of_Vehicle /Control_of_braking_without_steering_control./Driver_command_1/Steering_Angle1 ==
  Demux : Demux  Tag=STV Demux  Outputs=2
  FromWs : FromWorkspace  Tag=STV FromWs  VariableName=tuvar  SampleTime=0  SigBuilderData=DataTag2  VnvData=DataTag3
  Imported_Signal 1 : Outport  Tag=STV Outport
  Signal 1 : Outport  Tag=STV Outport  Port=2
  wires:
  Demux/2 -> Signal 1/1
  Demux/1 -> Imported_Signal 1/1
  FromWs/1 -> Demux/1

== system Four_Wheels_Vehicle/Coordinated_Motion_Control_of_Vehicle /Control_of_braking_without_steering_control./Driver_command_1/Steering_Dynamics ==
  Driver Torque : Inport
  Add : Sum  Inputs=+---
  Gain : Gain  Gain=25
  Gain1 : Gain  Gain=0.0065
  Gain2 : Gain  Gain=360/(2*pi)
  Gain3 : Gain  Gain=115
  Gain5 : Gain  Gain=2
  Gain6 : Gain  Gain=0.361
  Integrator : Integrator
  Integrator1 : Integrator
  Saturation : Saturate  UpperLimit=1  LowerLimit=-1
  Scope{1..5,8,10} (7 alike) : Scope
  Sign1 : Signum
  Steering Wheel Angle : Outport
  Ts : Outport  Port=2
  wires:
  Saturation/1 -> Gain1/1
  Integrator/1 -> Scope4/1, Gain6/1, Integrator1/1
  Gain6/1 -> Gain5/1
  Gain1/1 -> Add/3, Scope3/1
  Gain5/1 -> Scope5/1, Add/4
  Gain3/1 -> Scope1/1, Add/2, Ts/1
  Gain2/1 -> Steering Wheel Angle/1, Scope2/1
  Driver Torque/1 -> Add/1, Scope10/1
  Add/1 -> Gain/1
  Gain/1 -> Integrator/1, Scope8/1
  Integrator1/1 -> Gain2/1, Gain3/1, Saturation/1, Sign1/1

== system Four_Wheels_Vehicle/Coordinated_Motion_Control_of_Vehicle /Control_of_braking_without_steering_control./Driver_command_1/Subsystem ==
  Product : Product
  Ramp : simulink/Sources/Ramp  slope=3  start=0  X0=0
  Scope : Scope
  Scope1 : Scope
  Trigonometric Function : Trigonometry
  Steering_Ang. : Outport
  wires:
  Product/1 -> Scope1/1, Steering_Ang./1
  Trigonometric Function/1 -> Scope/1, Product/2
  Ramp/1 -> Trigonometric Function/1, Product/1

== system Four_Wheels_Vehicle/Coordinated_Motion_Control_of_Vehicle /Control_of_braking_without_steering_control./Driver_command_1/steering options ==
  (+) bias --> RH turn (-) bias --> LH turn1 : Constant  Value=0.5
  (+) bias --> RH turn (-) bias --> LH turn2 : Constant  Value=0.5
  Display{,1..3} (4 alike) : Display
  Gain : Gain  Gain=0.5
  Gain1 : Gain  Gain=-0.5
  Gain{2..5} (4 alike) : Gain
  Multiport Switch : MultiPortSwitch
  Sum{,1..3} (4 alike) : Sum  Inputs=|++
  left turn? : ManualSwitch  CurrentSetting=0
  restart point for: data received average1 : Constant
  restart point for: data received average2 : Constant  Value=0
  restart point for: data received average3 : Constant
  restart point for: data received average4 : Constant  Value=0
  right turn? : ManualSwitch  CurrentSetting=0
  steer select : Constant  Value=3
  turn LEFT hard : Step  Time=10  After=-1  SampleTime=0
  turn LEFT medium : Step  Time=30  After=-0.5  SampleTime=0
  turn RIGHT hard : Step  Time=20  After=+1  SampleTime=0
  delta_steer (rad) : Outport
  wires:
  Gain5/1 -> Sum1/1
  Gain4/1 -> Sum2/2, Display1/1
  Gain3/1 -> Sum2/1
  Gain2/1 -> Sum3/1
  Sum3/1 -> Sum1/2, Display3/1
  Sum2/1 -> Sum3/2, Display2/1
  turn LEFT hard/1 -> Gain2/1
  turn LEFT medium/1 -> Gain4/1
  turn RIGHT hard/1 -> Gain3/1
  (+) bias --> RH turn (-) bias --> LH turn1/1 -> Gain5/1
  Sum1/1 -> Display/1, Multiport Switch/4
  Gain1/1 -> Sum/2
  Gain/1 -> Sum/1
  left turn?/1 -> Gain1/1
  restart point for: data received average4/1 -> left turn?/2
  restart point for: data received average3/1 -> left turn?/1
  right turn?/1 -> Gain/1
  Sum/1 -> Multiport Switch/3
  restart point for: data received average2/1 -> right turn?/2
  restart point for: data received average1/1 -> right turn?/1
  Multiport Switch/1 -> delta_steer (rad)/1
  steer select/1 -> Multiport Switch/1
  (+) bias --> RH turn (-) bias --> LH turn2/1 -> Multiport Switch/2  "delta_steer (rad)"

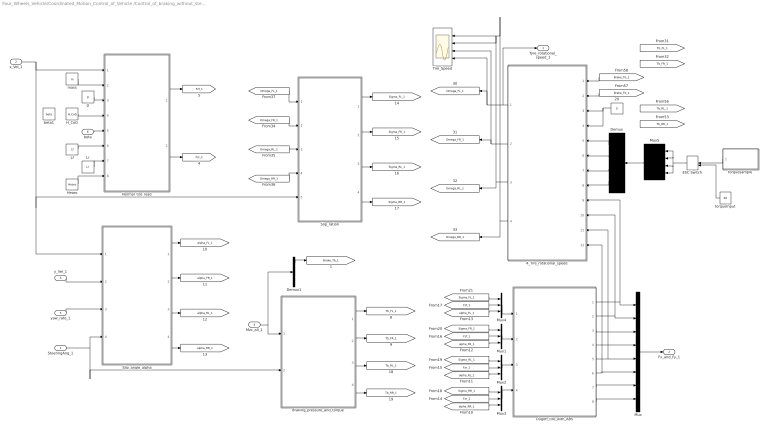
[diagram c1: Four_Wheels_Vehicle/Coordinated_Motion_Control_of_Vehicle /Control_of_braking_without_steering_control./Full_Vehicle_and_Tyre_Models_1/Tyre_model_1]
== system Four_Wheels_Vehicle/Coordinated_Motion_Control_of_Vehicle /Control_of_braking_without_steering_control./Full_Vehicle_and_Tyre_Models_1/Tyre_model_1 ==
  SteeringAng_1 : Inport
  x_Vel_1 : Inport  Port=2
  y_Vel_1 : Inport  Port=3
  Mzc_all_1 : Inport  Port=4
  yaw_rate_1 : Inport  Port=5
  beta : Inport  Port=6
  20 : Constant  Value=0
  4_Tire_rotational_speed : Subsystem
  Braking_pressure_and_torque : Subsystem
  Demux : Demux
  Demux1 : Demux
  Dugoff_tire_with_ABS : Subsystem
  ESC Switch : ManualSwitch
  H_CoG : Constant  Value=H_CoG
  Hearo : Constant  Value=Hearo
  Lf : Constant  Value=Lf
  Lr : Constant  Value=Lr
  Mux : Mux  Inputs=8
  Mux{1..4} (4 alike) : Mux  Inputs=3
  Mux5 : Mux
  Normal_tire_load : Subsystem
  Slip_angle_alpha : Subsystem
  Slip_ration : Subsystem
  Tire_Speed : Scope  NumInputPorts=4
  beta1 : Constant  Value=beta
  g : Constant  Value=g
  mass : Constant  Value=m
  torqueInput : Constant  Value=50
  "torquesample " : Subsystem  Tag=STV Subsys  LoadFcn=sigbuilder_block('load');  StartFcn=sigbuilder_block('start');  StopFcn=sigbuilder_block('stop');  ClipboardFcn=sigbuilder_block('clipboard');
  Tyre_rotational_speed_1 : Outport
  Fx_and_Fy_1 : Outport  Port=2
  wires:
  Mux/1 -> Fx_and_Fy_1/1
  Dugoff_tire_with_ABS/3(Fy_FL_1) -> Mux/3
  Dugoff_tire_with_ABS/4(Fy_FR_1) -> Mux/4
  Dugoff_tire_with_ABS/7(Fy_RL_1) -> Mux/7
  Dugoff_tire_with_ABS/8(Fy_RR_1) -> Mux/8
  Slip_angle_alpha/2(alpha_FR_1) -> [alpha_FR_1]
  Slip_angle_alpha/1(alpha_FL_1) -> [alpha_FL_1]
  Slip_angle_alpha/3(alpha_RL_1) -> [alpha_RL_1]
  [Fzf_1] -> Mux1/2
  [Fzr_1] -> Mux2/2
  Normal_tire_load/1(Fz_f_1) -> [Fzf_1]
  [Brake_Tb_1] -> 4_Tire_rotational_speed/2(Tb_FR_1)
  [Brake_Tb_1] -> 4_Tire_rotational_speed/1(Tb_FL_1)
  [Fzr_1] -> Mux3/2
  4_Tire_rotational_speed/4(Omega_RR_1) -> [Omega_RR_1], Tire_Speed/1
  20/1 -> 4_Tire_rotational_speed/3(Tb_RL_1), 4_Tire_rotational_speed/4(Tb_RR_1)
  [Fzf_1] -> Mux4/2
  Slip_angle_alpha/4(alpha_RR_1) -> [alpha_RR_1]
  torqueInput/1 -> ESC Switch/2
  Demux/1 -> 4_Tire_rotational_speed/5(Td_FL_1)
  g/1 -> Normal_tire_load/3(g)
  Hearo/1 -> Normal_tire_load/8(Hearo)
  Normal_tire_load/2(Fz_r_1) -> [Fzr_1]
  4_Tire_rotational_speed/2(Omega_FR_1) -> [Omega_FR_1], Tire_Speed/3
  [Sigma_FL_1] -> Mux4/1
  mass/1 -> Normal_tire_load/2(mass)
  beta/1 -> Normal_tire_load/5(beta)
  Dugoff_tire_with_ABS/1(Fx_FL_1) -> 4_Tire_rotational_speed/9(Fx_FL_1), Mux/1
  [Sigma_RR_1] -> Mux3/1
  Dugoff_tire_with_ABS/2(Fx_FR_1) -> 4_Tire_rotational_speed/10(Fx_FR_1), Mux/2
  [Omega_RL_1] -> Slip_ration/3(Omega_RL_1)
  x_Vel_1/1 -> Normal_tire_load/1(x_Vel_1), Slip_ration/5(x_Vel_1), Slip_angle_alpha/1(x_Vel_1)
  [Sigma_FR_1] -> Mux1/1
  [Omega_RR_1] -> Slip_ration/4(Omega_RR_1)
  [Omega_FL_1] -> Slip_ration/1(Omega_FL_1)
  Demux/4 -> 4_Tire_rotational_speed/8(Td_RR_1)
  [alpha_FL_1] -> Mux4/3
  Dugoff_tire_with_ABS/6(Fx_RR_1) -> 4_Tire_rotational_speed/12(Fx_RR_1), Mux/6
  [alpha_FR_1] -> Mux1/3
  Demux/3 -> 4_Tire_rotational_speed/7(Td_RL_1)
  [Omega_FR_1] -> Slip_ration/2(Omega_FR_1)
  ESC Switch/1 -> Mux5/2, Mux5/1, Mux5/3, Mux5/4
  Mux5/1 -> Demux/1
  4_Tire_rotational_speed/3(Omega_RL_1) -> [Omega_RL_1], Tire_Speed/2
  H_CoG/1 -> Normal_tire_load/4(H_CoG)
  Lf/1 -> Normal_tire_load/6(Lf)
  [Sigma_RL_1] -> Mux2/1
  SteeringAng_1/1 -> Slip_angle_alpha/4(Steering_Ang._1), Braking_pressure_and_torque/2(SteeringAng)
  Dugoff_tire_with_ABS/5(Fx_RL_1) -> 4_Tire_rotational_speed/11(Fx_RL_1), Mux/5
  "torquesample "/1(Signal 1) -> ESC Switch/1
  Demux/2 -> 4_Tire_rotational_speed/6(Td_FR_1)
  4_Tire_rotational_speed/1(Omega_FL_1) -> [Omega_FL_1], Tire_Speed/4, Tyre_rotational_speed_1/1
  Lr/1 -> Normal_tire_load/7(Lr)
  Slip_ration/2(Sigma_FR_1) -> [Sigma_FR_1]
  [alpha_RR_1] -> Mux3/3
  Mux4/1 -> Dugoff_tire_with_ABS/1(In1)
  Mux1/1 -> Dugoff_tire_with_ABS/2(In2)
  Mux3/1 -> Dugoff_tire_with_ABS/4(In3)
  Slip_ration/1(Sigma_FL_1) -> [Sigma_FL_1]
  Slip_ration/3(Sigma_RL_1) -> [Sigma_RL_1]
  y_Vel_1/1 -> Slip_angle_alpha/2(y_Vel_1)
  Mux2/1 -> Dugoff_tire_with_ABS/3(In5)
  [alpha_RL_1] -> Mux2/3
  Slip_ration/4(Sigma_RR_1) -> [Sigma_RR_1]
  yaw_rate_1/1 -> Slip_angle_alpha/3(yaw_rate_1)
  Braking_pressure_and_torque/3(Tb_RL_1) -> [Tb_RL_1]
  Braking_pressure_and_torque/2(Tb_FR_1) -> [Tb_FR_1]
  Braking_pressure_and_torque/1(Tb_FL_1) -> [Tb_FL_1]
  Braking_pressure_and_torque/4(Tb_RR_1) -> [Tb_RR_1]
  Mzc_all_1/1 -> Demux1/1, Braking_pressure_and_torque/1(Mzc_all_1)
  Demux1/1 -> [Brake_Tb_1]
